FUNCTION_BLOCK "IMAC_VALVE_CALL"
TITLE =Function calls for VALVE objects
//Parameter Description for Function VALVE (FB83):
//-------------------------------------------------
//OBJ:     Ascending Object number for VALVE (1...x)
//
//RMOT:    'REMOTE'     Feedback
//                      0 = Local
//                      1 = Remote
//
//OPEN:    'OPEN'       Feedback
//                      0 = Valve is not OPEN
//                      1 = Valve is OPEN
//
//CLSD:    'CLOSED'     Feedback
//                      0 = Valve is not CLOSED
//                      1 = Valve is CLOSED
//
//ACOM:    'AUTO' Mode  Command Interface (only active, if 'REMOTE'+'AUTO')
//                      Bit  8       : Open  Command
//                      Bit  9       : Close Command
//                      Bit 11       : Lock 'Open / Close'
//                      Bit 12       : Emergency Close Command
//                      Bit 13       : Blackout Start Command
//                      Bit 14       : Pleiger 24V Valve (special function)
//
//FAUL:    'EXT. FAULT' Feedback. Function dep. on Mode Switch 'M10_ExtFaultNC':
//                      If 'M10_ExtFaultNC' = 0 :   0 = OK,    1 = Fault
//                      If 'M10_ExtFaultNC' = 1 :   0 = Fault, 1 = OK
//
//PCONF:   (leave empty, refers to local instance data in Instance DB)
//
//VOPN:    'OPEN'       Output to Valve
//                      0 = No Command
//                      1 = Open Command
//
//VCLS:    'CLOSE'      Output to Valve
//                      0 = No Command
//                      1 = Close Command
//
//STAT:    'AUTO' Mode  Status Interface
//                      Bit  8       : Valve Status Opened
//                      Bit  9       : Valve Status Closed
//                      Bit 10       : Local
//                      Bit 11       : Manual
//                      Bit 12       : Auto
//                      Bit 13       : Valve Opening
//                      Bit 14       : Valve Closing
//                      Bit 15       : Valve Alarm
//
//OSSTAT:  OS Status Word
//                      Value = 0    : Undefined
//                      Value = 1    : Opened
//                      Value = 2    : Closed
//                      Value = 3    : Opening
//                      Value = 4    : Closing
//                      Value = 5    : Undefined Position
//                      Value + 256  : Local Mode  (Offset Value)
//                      Value + 512  : Manual Mode (Offset Value)
//                      Value + 1024 : Auto Mode   (Offset Value)
//
//OSALARM: OS Alarm Word
//                      Value = 0    : Undefined
//                      Value = 1    : Normal
//                      Value = 2    : External Fault Alarm
//                      Value = 3    : Moving Alarm
//                      Value = 4    : Opening Alarm
//                      Value = 5    : Closing Alarm
//                      Value = 6    : Non-Feedback Alarm
//                      Value = 7    : Lock Start / Stop Commands
//                      Value = 8    : Emergency Off
//
//OSCOM:   OS Command Interface
//                      Bit  0       : Open   Command
//                      Bit  1       : Close  Command
//                      Bit  2       : Toggle Command
//                      Bit  7       : Reset  Command
//                      Bit  9       : Manual Command
//                      Bit 10       : Auto   Command
AUTHOR : Hottendo
FAMILY : IMAC
VERSION : 0.2


VAR
  ValveNo_001 : "IMAC_VALVE";
  ValveNo_002 : "IMAC_VALVE";
  ValveNo_003 : "IMAC_VALVE";
  ValveNo_004 : "IMAC_VALVE";
  ValveNo_005 : "IMAC_VALVE";
  ValveNo_006 : "IMAC_VALVE";
  ValveNo_007 : "IMAC_VALVE";
  ValveNo_008 : "IMAC_VALVE";
  ValveNo_009 : "IMAC_VALVE";
  ValveNo_010 : "IMAC_VALVE";
  ValveNo_011 : "IMAC_VALVE";
  ValveNo_012 : "IMAC_VALVE";
  ValveNo_013 : "IMAC_VALVE";
  ValveNo_014 : "IMAC_VALVE";
  ValveNo_015 : "IMAC_VALVE";
  ValveNo_016 : "IMAC_VALVE";
  ValveNo_017 : "IMAC_VALVE";
  ValveNo_018 : "IMAC_VALVE";
  ValveNo_019 : "IMAC_VALVE";
  ValveNo_020 : "IMAC_VALVE";
  ValveNo_021 : "IMAC_VALVE";
  ValveNo_022 : "IMAC_VALVE";
  ValveNo_023 : "IMAC_VALVE";
  ValveNo_024 : "IMAC_VALVE";
  ValveNo_025 : "IMAC_VALVE";
  ValveNo_026 : "IMAC_VALVE";
  ValveNo_027 : "IMAC_VALVE";
  ValveNo_028 : "IMAC_VALVE";
  ValveNo_029 : "IMAC_VALVE";
  ValveNo_030 : "IMAC_VALVE";
  ValveNo_031 : "IMAC_VALVE";
  ValveNo_032 : "IMAC_VALVE";
  ValveNo_033 : "IMAC_VALVE";
  ValveNo_034 : "IMAC_VALVE";
  ValveNo_035 : "IMAC_VALVE";
  ValveNo_036 : "IMAC_VALVE";
  ValveNo_037 : "IMAC_VALVE";
  ValveNo_038 : "IMAC_VALVE";
  ValveNo_039 : "IMAC_VALVE";
  ValveNo_040 : "IMAC_VALVE";
  ValveNo_041 : "IMAC_VALVE";
  ValveNo_042 : "IMAC_VALVE";
  ValveNo_043 : "IMAC_VALVE";
  ValveNo_044 : "IMAC_VALVE";
  ValveNo_045 : "IMAC_VALVE";
  ValveNo_046 : "IMAC_VALVE";
  ValveNo_047 : "IMAC_VALVE";
  ValveNo_048 : "IMAC_VALVE";
  ValveNo_049 : "IMAC_VALVE";
  ValveNo_050 : "IMAC_VALVE";
  ValveNo_051 : "IMAC_VALVE";
  ValveNo_052 : "IMAC_VALVE";
  ValveNo_053 : "IMAC_VALVE";
  ValveNo_054 : "IMAC_VALVE";
  ValveNo_055 : "IMAC_VALVE";
  ValveNo_056 : "IMAC_VALVE";
  ValveNo_057 : "IMAC_VALVE";
  ValveNo_058 : "IMAC_VALVE";
  ValveNo_059 : "IMAC_VALVE";
  ValveNo_060 : "IMAC_VALVE";
  ValveNo_061 : "IMAC_VALVE";
  ValveNo_062 : "IMAC_VALVE";
  ValveNo_063 : "IMAC_VALVE";
  ValveNo_064 : "IMAC_VALVE";
  ValveNo_065 : "IMAC_VALVE";
  ValveNo_066 : "IMAC_VALVE";
  ValveNo_067 : "IMAC_VALVE";
  ValveNo_068 : "IMAC_VALVE";
  ValveNo_069 : "IMAC_VALVE";
  ValveNo_070 : "IMAC_VALVE";
  ValveNo_071 : "IMAC_VALVE";
  ValveNo_072 : "IMAC_VALVE";
  ValveNo_073 : "IMAC_VALVE";
  ValveNo_074 : "IMAC_VALVE";
  ValveNo_075 : "IMAC_VALVE";
  ValveNo_076 : "IMAC_VALVE";
  ValveNo_077 : "IMAC_VALVE";
  ValveNo_078 : "IMAC_VALVE";
  ValveNo_079 : "IMAC_VALVE";
  ValveNo_080 : "IMAC_VALVE";
  ValveNo_081 : "IMAC_VALVE";
  ValveNo_082 : "IMAC_VALVE";
  ValveNo_083 : "IMAC_VALVE";
  ValveNo_084 : "IMAC_VALVE";
  ValveNo_085 : "IMAC_VALVE";
  ValveNo_086 : "IMAC_VALVE";
  ValveNo_087 : "IMAC_VALVE";
  ValveNo_088 : "IMAC_VALVE";
  ValveNo_089 : "IMAC_VALVE";
  ValveNo_090 : "IMAC_VALVE";
  ValveNo_091 : "IMAC_VALVE";
  ValveNo_092 : "IMAC_VALVE";
  ValveNo_093 : "IMAC_VALVE";
  ValveNo_094 : "IMAC_VALVE";
  ValveNo_095 : "IMAC_VALVE";
  ValveNo_096 : "IMAC_VALVE";
  ValveNo_097 : "IMAC_VALVE";
  ValveNo_098 : "IMAC_VALVE";
  ValveNo_099 : "IMAC_VALVE";
  ValveNo_100 : "IMAC_VALVE";
END_VAR
BEGIN
NETWORK
TITLE =VALVE Number 001

      CALL #ValveNo_001 (
           OBJ                      := 1,
           RMOT                     := E      7.6,
           OPEN                     := E      7.7,
           CLSD                     := E      8.0,
           ACOM                     := "IMAC_VALVE_I/O".VALVE_001_ACOM,
           FAUL                     := E      8.1,
           VOPN                     := A      3.6,
           VCLS                     := A      3.7,
           STAT                     := "IMAC_VALVE_I/O".VALVE_001_STAT,
           OSSTAT                   := "IMAC_VALVE_I/O".VALVE_00l_OSSTAT,
           OSALARM                  := "IMAC_VALVE_I/O".VALVE_00l_OSALARM,
           OSCOM                    := "IMAC_VALVE_I/O".VALVE_001_OSCOM);

NETWORK
TITLE =VALVE Number 002

      CALL #ValveNo_002 (
           OBJ                      := 2,
           RMOT                     := E      8.2,
           OPEN                     := E      8.3,
           CLSD                     := E      8.4,
           ACOM                     := "IMAC_VALVE_I/O".VALVE_002_ACOM,
           FAUL                     := E      8.5,
           VOPN                     := A      4.0,
           VCLS                     := A      4.1,
           STAT                     := "IMAC_VALVE_I/O".VALVE_002_STAT,
           OSSTAT                   := "IMAC_VALVE_I/O".VALVE_002_OSSTAT,
           OSALARM                  := "IMAC_VALVE_I/O".VALVE_002_OSALARM,
           OSCOM                    := "IMAC_VALVE_I/O".VALVE_002_OSCOM);

NETWORK
TITLE =VALVE Number 003

      CALL #ValveNo_003 (
           OBJ                      := 3,
           RMOT                     := E      8.6,
           OPEN                     := E      8.7,
           CLSD                     := E      9.0,
           ACOM                     := "IMAC_VALVE_I/O".VALVE_003_ACOM,
           FAUL                     := E      9.1,
           VOPN                     := A      4.2,
           VCLS                     := A      4.3,
           STAT                     := "IMAC_VALVE_I/O".VALVE_003_STAT,
           OSSTAT                   := "IMAC_VALVE_I/O".VALVE_003_OSSTAT,
           OSALARM                  := "IMAC_VALVE_I/O".VALVE_003_OSALARM,
           OSCOM                    := "IMAC_VALVE_I/O".VALVE_003_OSCOM);

NETWORK
TITLE =VALVE Number 004

//*********** END of Function Processing ! *******************************************************************
      BEA   ; // Move this Instruction down to the next Network to add one object !
//************************************************************************************************************

      CALL #ValveNo_004 (
           OBJ                      := 4,
           ACOM                     := "IMAC_VALVE_I/O".VALVE_004_ACOM,
           STAT                     := "IMAC_VALVE_I/O".VALVE_004_STAT,
           OSSTAT                   := "IMAC_VALVE_I/O".VALVE_004_OSSTAT,
           OSALARM                  := "IMAC_VALVE_I/O".VALVE_004_OSALARM,
           OSCOM                    := "IMAC_VALVE_I/O".VALVE_004_OSCOM);

NETWORK
TITLE =VALVE Number 005

      CALL #ValveNo_005 (
           OBJ                      := 5,
           ACOM                     := "IMAC_VALVE_I/O".VALVE_005_ACOM,
           STAT                     := "IMAC_VALVE_I/O".VALVE_005_STAT,
           OSSTAT                   := "IMAC_VALVE_I/O".VALVE_005_OSSTAT,
           OSALARM                  := "IMAC_VALVE_I/O".VALVE_005_OSALARM,
           OSCOM                    := "IMAC_VALVE_I/O".VALVE_005_OSCOM);

NETWORK
TITLE =VALVE Number 006

      CALL #ValveNo_006 (
           OBJ                      := 6,
           ACOM                     := "IMAC_VALVE_I/O".VALVE_006_ACOM,
           STAT                     := "IMAC_VALVE_I/O".VALVE_006_STAT,
           OSSTAT                   := "IMAC_VALVE_I/O".VALVE_006_OSSTAT,
           OSALARM                  := "IMAC_VALVE_I/O".VALVE_006_OSALARM,
           OSCOM                    := "IMAC_VALVE_I/O".VALVE_006_OSCOM);

NETWORK
TITLE =VALVE Number 007

      CALL #ValveNo_007 (
           OBJ                      := 7,
           ACOM                     := "IMAC_VALVE_I/O".VALVE_007_ACOM,
           STAT                     := "IMAC_VALVE_I/O".VALVE_007_STAT,
           OSSTAT                   := "IMAC_VALVE_I/O".VALVE_007_OSSTAT,
           OSALARM                  := "IMAC_VALVE_I/O".VALVE_007_OSALARM,
           OSCOM                    := "IMAC_VALVE_I/O".VALVE_007_OSCOM);

NETWORK
TITLE =VALVE Number 008

      CALL #ValveNo_008 (
           OBJ                      := 8,
           ACOM                     := "IMAC_VALVE_I/O".VALVE_008_ACOM,
           STAT                     := "IMAC_VALVE_I/O".VALVE_008_STAT,
           OSSTAT                   := "IMAC_VALVE_I/O".VALVE_008_OSSTAT,
           OSALARM                  := "IMAC_VALVE_I/O".VALVE_008_OSALARM,
           OSCOM                    := "IMAC_VALVE_I/O".VALVE_008_OSCOM);

NETWORK
TITLE =VALVE Number 009

      CALL #ValveNo_009 (
           OBJ                      := 9,
           ACOM                     := "IMAC_VALVE_I/O".VALVE_009_ACOM,
           STAT                     := "IMAC_VALVE_I/O".VALVE_009_STAT,
           OSSTAT                   := "IMAC_VALVE_I/O".VALVE_009_OSSTAT,
           OSALARM                  := "IMAC_VALVE_I/O".VALVE_009_OSALARM,
           OSCOM                    := "IMAC_VALVE_I/O".VALVE_009_OSCOM);

NETWORK
TITLE =VALVE Number 010

      CALL #ValveNo_010 (
           OBJ                      := 10,
           ACOM                     := "IMAC_VALVE_I/O".VALVE_010_ACOM,
           STAT                     := "IMAC_VALVE_I/O".VALVE_010_STAT,
           OSSTAT                   := "IMAC_VALVE_I/O".VALVE_010_OSSTAT,
           OSALARM                  := "IMAC_VALVE_I/O".VALVE_010_OSALARM,
           OSCOM                    := "IMAC_VALVE_I/O".VALVE_010_OSCOM);

NETWORK
TITLE =VALVE Number 011

//*********** END of Function Processing ! *******************************************************************
      BEA   ; // Move this Instruction down to the next Network to add one object !
//************************************************************************************************************

      CALL #ValveNo_011 (
           OBJ                      := 11,
           ACOM                     := "IMAC_VALVE_I/O".VALVE_011_ACOM,
           STAT                     := "IMAC_VALVE_I/O".VALVE_011_STAT,
           OSSTAT                   := "IMAC_VALVE_I/O".VALVE_01l_OSSTAT,
           OSALARM                  := "IMAC_VALVE_I/O".VALVE_01l_OSALARM,
           OSCOM                    := "IMAC_VALVE_I/O".VALVE_011_OSCOM);

NETWORK
TITLE =VALVE Number 012

      CALL #ValveNo_012 (
           OBJ                      := 12,
           ACOM                     := "IMAC_VALVE_I/O".VALVE_012_ACOM,
           STAT                     := "IMAC_VALVE_I/O".VALVE_012_STAT,
           OSSTAT                   := "IMAC_VALVE_I/O".VALVE_012_OSSTAT,
           OSALARM                  := "IMAC_VALVE_I/O".VALVE_012_OSALARM,
           OSCOM                    := "IMAC_VALVE_I/O".VALVE_012_OSCOM);

NETWORK
TITLE =VALVE Number 013

      CALL #ValveNo_013 (
           OBJ                      := 13,
           ACOM                     := "IMAC_VALVE_I/O".VALVE_013_ACOM,
           STAT                     := "IMAC_VALVE_I/O".VALVE_013_STAT,
           OSSTAT                   := "IMAC_VALVE_I/O".VALVE_013_OSSTAT,
           OSALARM                  := "IMAC_VALVE_I/O".VALVE_013_OSALARM,
           OSCOM                    := "IMAC_VALVE_I/O".VALVE_013_OSCOM);

NETWORK
TITLE =VALVE Number 014

      CALL #ValveNo_014 (
           OBJ                      := 14,
           ACOM                     := "IMAC_VALVE_I/O".VALVE_014_ACOM,
           STAT                     := "IMAC_VALVE_I/O".VALVE_014_STAT,
           OSSTAT                   := "IMAC_VALVE_I/O".VALVE_014_OSSTAT,
           OSALARM                  := "IMAC_VALVE_I/O".VALVE_014_OSALARM,
           OSCOM                    := "IMAC_VALVE_I/O".VALVE_014_OSCOM);

NETWORK
TITLE =VALVE Number 015

      CALL #ValveNo_015 (
           OBJ                      := 15,
           ACOM                     := "IMAC_VALVE_I/O".VALVE_015_ACOM,
           STAT                     := "IMAC_VALVE_I/O".VALVE_015_STAT,
           OSSTAT                   := "IMAC_VALVE_I/O".VALVE_015_OSSTAT,
           OSALARM                  := "IMAC_VALVE_I/O".VALVE_015_OSALARM,
           OSCOM                    := "IMAC_VALVE_I/O".VALVE_015_OSCOM);

NETWORK
TITLE =VALVE Number 016

      CALL #ValveNo_016 (
           OBJ                      := 16,
           ACOM                     := "IMAC_VALVE_I/O".VALVE_016_ACOM,
           STAT                     := "IMAC_VALVE_I/O".VALVE_016_STAT,
           OSSTAT                   := "IMAC_VALVE_I/O".VALVE_016_OSSTAT,
           OSALARM                  := "IMAC_VALVE_I/O".VALVE_016_OSALARM,
           OSCOM                    := "IMAC_VALVE_I/O".VALVE_016_OSCOM);

NETWORK
TITLE =VALVE Number 017

      CALL #ValveNo_017 (
           OBJ                      := 17,
           ACOM                     := "IMAC_VALVE_I/O".VALVE_017_ACOM,
           STAT                     := "IMAC_VALVE_I/O".VALVE_017_STAT,
           OSSTAT                   := "IMAC_VALVE_I/O".VALVE_017_OSSTAT,
           OSALARM                  := "IMAC_VALVE_I/O".VALVE_017_OSALARM,
           OSCOM                    := "IMAC_VALVE_I/O".VALVE_017_OSCOM);

NETWORK
TITLE =VALVE Number 018

      CALL #ValveNo_018 (
           OBJ                      := 18,
           ACOM                     := "IMAC_VALVE_I/O".VALVE_018_ACOM,
           STAT                     := "IMAC_VALVE_I/O".VALVE_018_STAT,
           OSSTAT                   := "IMAC_VALVE_I/O".VALVE_018_OSSTAT,
           OSALARM                  := "IMAC_VALVE_I/O".VALVE_018_OSALARM,
           OSCOM                    := "IMAC_VALVE_I/O".VALVE_018_OSCOM);

NETWORK
TITLE =VALVE Number 019

      CALL #ValveNo_019 (
           OBJ                      := 19,
           ACOM                     := "IMAC_VALVE_I/O".VALVE_019_ACOM,
           STAT                     := "IMAC_VALVE_I/O".VALVE_019_STAT,
           OSSTAT                   := "IMAC_VALVE_I/O".VALVE_019_OSSTAT,
           OSALARM                  := "IMAC_VALVE_I/O".VALVE_019_OSALARM,
           OSCOM                    := "IMAC_VALVE_I/O".VALVE_019_OSCOM);

NETWORK
TITLE =VALVE Number 020

      CALL #ValveNo_020 (
           OBJ                      := 20,
           ACOM                     := "IMAC_VALVE_I/O".VALVE_020_ACOM,
           STAT                     := "IMAC_VALVE_I/O".VALVE_020_STAT,
           OSSTAT                   := "IMAC_VALVE_I/O".VALVE_020_OSSTAT,
           OSALARM                  := "IMAC_VALVE_I/O".VALVE_020_OSALARM,
           OSCOM                    := "IMAC_VALVE_I/O".VALVE_020_OSCOM);

NETWORK
TITLE =VALVE Number 021

      CALL #ValveNo_021 (
           OBJ                      := 21,
           ACOM                     := "IMAC_VALVE_I/O".VALVE_021_ACOM,
           STAT                     := "IMAC_VALVE_I/O".VALVE_021_STAT,
           OSSTAT                   := "IMAC_VALVE_I/O".VALVE_02l_OSSTAT,
           OSALARM                  := "IMAC_VALVE_I/O".VALVE_02l_OSALARM,
           OSCOM                    := "IMAC_VALVE_I/O".VALVE_021_OSCOM);

NETWORK
TITLE =VALVE Number 022

      CALL #ValveNo_022 (
           OBJ                      := 22,
           ACOM                     := "IMAC_VALVE_I/O".VALVE_022_ACOM,
           STAT                     := "IMAC_VALVE_I/O".VALVE_022_STAT,
           OSSTAT                   := "IMAC_VALVE_I/O".VALVE_022_OSSTAT,
           OSALARM                  := "IMAC_VALVE_I/O".VALVE_022_OSALARM,
           OSCOM                    := "IMAC_VALVE_I/O".VALVE_022_OSCOM);

NETWORK
TITLE =VALVE Number 023

      CALL #ValveNo_023 (
           OBJ                      := 23,
           ACOM                     := "IMAC_VALVE_I/O".VALVE_023_ACOM,
           STAT                     := "IMAC_VALVE_I/O".VALVE_023_STAT,
           OSSTAT                   := "IMAC_VALVE_I/O".VALVE_023_OSSTAT,
           OSALARM                  := "IMAC_VALVE_I/O".VALVE_023_OSALARM,
           OSCOM                    := "IMAC_VALVE_I/O".VALVE_023_OSCOM);

NETWORK
TITLE =VALVE Number 024

      CALL #ValveNo_024 (
           OBJ                      := 24,
           ACOM                     := "IMAC_VALVE_I/O".VALVE_024_ACOM,
           STAT                     := "IMAC_VALVE_I/O".VALVE_024_STAT,
           OSSTAT                   := "IMAC_VALVE_I/O".VALVE_024_OSSTAT,
           OSALARM                  := "IMAC_VALVE_I/O".VALVE_024_OSALARM,
           OSCOM                    := "IMAC_VALVE_I/O".VALVE_024_OSCOM);

NETWORK
TITLE =VALVE Number 025

      CALL #ValveNo_025 (
           OBJ                      := 25,
           ACOM                     := "IMAC_VALVE_I/O".VALVE_025_ACOM,
           STAT                     := "IMAC_VALVE_I/O".VALVE_025_STAT,
           OSSTAT                   := "IMAC_VALVE_I/O".VALVE_025_OSSTAT,
           OSALARM                  := "IMAC_VALVE_I/O".VALVE_025_OSALARM,
           OSCOM                    := "IMAC_VALVE_I/O".VALVE_025_OSCOM);

NETWORK
TITLE =VALVE Number 026

      CALL #ValveNo_026 (
           OBJ                      := 26,
           ACOM                     := "IMAC_VALVE_I/O".VALVE_026_ACOM,
           STAT                     := "IMAC_VALVE_I/O".VALVE_026_STAT,
           OSSTAT                   := "IMAC_VALVE_I/O".VALVE_026_OSSTAT,
           OSALARM                  := "IMAC_VALVE_I/O".VALVE_026_OSALARM,
           OSCOM                    := "IMAC_VALVE_I/O".VALVE_026_OSCOM);

NETWORK
TITLE =VALVE Number 027

      CALL #ValveNo_027 (
           OBJ                      := 27,
           ACOM                     := "IMAC_VALVE_I/O".VALVE_027_ACOM,
           STAT                     := "IMAC_VALVE_I/O".VALVE_027_STAT,
           OSSTAT                   := "IMAC_VALVE_I/O".VALVE_027_OSSTAT,
           OSALARM                  := "IMAC_VALVE_I/O".VALVE_027_OSALARM,
           OSCOM                    := "IMAC_VALVE_I/O".VALVE_027_OSCOM);

NETWORK
TITLE =VALVE Number 028

      CALL #ValveNo_028 (
           OBJ                      := 28,
           ACOM                     := "IMAC_VALVE_I/O".VALVE_028_ACOM,
           STAT                     := "IMAC_VALVE_I/O".VALVE_028_STAT,
           OSSTAT                   := "IMAC_VALVE_I/O".VALVE_028_OSSTAT,
           OSALARM                  := "IMAC_VALVE_I/O".VALVE_028_OSALARM,
           OSCOM                    := "IMAC_VALVE_I/O".VALVE_028_OSCOM);

NETWORK
TITLE =VALVE Number 029

      CALL #ValveNo_029 (
           OBJ                      := 29,
           ACOM                     := "IMAC_VALVE_I/O".VALVE_029_ACOM,
           STAT                     := "IMAC_VALVE_I/O".VALVE_029_STAT,
           OSSTAT                   := "IMAC_VALVE_I/O".VALVE_029_OSSTAT,
           OSALARM                  := "IMAC_VALVE_I/O".VALVE_029_OSALARM,
           OSCOM                    := "IMAC_VALVE_I/O".VALVE_029_OSCOM);

NETWORK
TITLE =VALVE Number 030

      CALL #ValveNo_030 (
           OBJ                      := 30,
           ACOM                     := "IMAC_VALVE_I/O".VALVE_030_ACOM,
           STAT                     := "IMAC_VALVE_I/O".VALVE_030_STAT,
           OSSTAT                   := "IMAC_VALVE_I/O".VALVE_030_OSSTAT,
           OSALARM                  := "IMAC_VALVE_I/O".VALVE_030_OSALARM,
           OSCOM                    := "IMAC_VALVE_I/O".VALVE_030_OSCOM);

NETWORK
TITLE =VALVE Number 031

      CALL #ValveNo_031 (
           OBJ                      := 31,
           ACOM                     := "IMAC_VALVE_I/O".VALVE_031_ACOM,
           STAT                     := "IMAC_VALVE_I/O".VALVE_031_STAT,
           OSSTAT                   := "IMAC_VALVE_I/O".VALVE_03l_OSSTAT,
           OSALARM                  := "IMAC_VALVE_I/O".VALVE_03l_OSALARM,
           OSCOM                    := "IMAC_VALVE_I/O".VALVE_031_OSCOM);

NETWORK
TITLE =VALVE Number 032

      CALL #ValveNo_032 (
           OBJ                      := 32,
           ACOM                     := "IMAC_VALVE_I/O".VALVE_032_ACOM,
           STAT                     := "IMAC_VALVE_I/O".VALVE_032_STAT,
           OSSTAT                   := "IMAC_VALVE_I/O".VALVE_032_OSSTAT,
           OSALARM                  := "IMAC_VALVE_I/O".VALVE_032_OSALARM,
           OSCOM                    := "IMAC_VALVE_I/O".VALVE_032_OSCOM);

NETWORK
TITLE =VALVE Number 033

      CALL #ValveNo_033 (
           OBJ                      := 33,
           ACOM                     := "IMAC_VALVE_I/O".VALVE_033_ACOM,
           STAT                     := "IMAC_VALVE_I/O".VALVE_033_STAT,
           OSSTAT                   := "IMAC_VALVE_I/O".VALVE_033_OSSTAT,
           OSALARM                  := "IMAC_VALVE_I/O".VALVE_033_OSALARM,
           OSCOM                    := "IMAC_VALVE_I/O".VALVE_033_OSCOM);

NETWORK
TITLE =VALVE Number 034

      CALL #ValveNo_034 (
           OBJ                      := 34,
           ACOM                     := "IMAC_VALVE_I/O".VALVE_034_ACOM,
           STAT                     := "IMAC_VALVE_I/O".VALVE_034_STAT,
           OSSTAT                   := "IMAC_VALVE_I/O".VALVE_034_OSSTAT,
           OSALARM                  := "IMAC_VALVE_I/O".VALVE_034_OSALARM,
           OSCOM                    := "IMAC_VALVE_I/O".VALVE_034_OSCOM);

NETWORK
TITLE =VALVE Number 035

      CALL #ValveNo_035 (
           OBJ                      := 35,
           ACOM                     := "IMAC_VALVE_I/O".VALVE_035_ACOM,
           STAT                     := "IMAC_VALVE_I/O".VALVE_035_STAT,
           OSSTAT                   := "IMAC_VALVE_I/O".VALVE_035_OSSTAT,
           OSALARM                  := "IMAC_VALVE_I/O".VALVE_035_OSALARM,
           OSCOM                    := "IMAC_VALVE_I/O".VALVE_035_OSCOM);

NETWORK
TITLE =VALVE Number 036

      CALL #ValveNo_036 (
           OBJ                      := 36,
           ACOM                     := "IMAC_VALVE_I/O".VALVE_036_ACOM,
           STAT                     := "IMAC_VALVE_I/O".VALVE_036_STAT,
           OSSTAT                   := "IMAC_VALVE_I/O".VALVE_036_OSSTAT,
           OSALARM                  := "IMAC_VALVE_I/O".VALVE_036_OSALARM,
           OSCOM                    := "IMAC_VALVE_I/O".VALVE_036_OSCOM);

NETWORK
TITLE =VALVE Number 037

      CALL #ValveNo_037 (
           OBJ                      := 37,
           ACOM                     := "IMAC_VALVE_I/O".VALVE_037_ACOM,
           STAT                     := "IMAC_VALVE_I/O".VALVE_037_STAT,
           OSSTAT                   := "IMAC_VALVE_I/O".VALVE_037_OSSTAT,
           OSALARM                  := "IMAC_VALVE_I/O".VALVE_037_OSALARM,
           OSCOM                    := "IMAC_VALVE_I/O".VALVE_037_OSCOM);

NETWORK
TITLE =VALVE Number 038

      CALL #ValveNo_038 (
           OBJ                      := 38,
           ACOM                     := "IMAC_VALVE_I/O".VALVE_038_ACOM,
           STAT                     := "IMAC_VALVE_I/O".VALVE_038_STAT,
           OSSTAT                   := "IMAC_VALVE_I/O".VALVE_038_OSSTAT,
           OSALARM                  := "IMAC_VALVE_I/O".VALVE_038_OSALARM,
           OSCOM                    := "IMAC_VALVE_I/O".VALVE_038_OSCOM);

NETWORK
TITLE =VALVE Number 039

      CALL #ValveNo_039 (
           OBJ                      := 339,
           ACOM                     := "IMAC_VALVE_I/O".VALVE_039_ACOM,
           STAT                     := "IMAC_VALVE_I/O".VALVE_039_STAT,
           OSSTAT                   := "IMAC_VALVE_I/O".VALVE_039_OSSTAT,
           OSALARM                  := "IMAC_VALVE_I/O".VALVE_039_OSALARM,
           OSCOM                    := "IMAC_VALVE_I/O".VALVE_039_OSCOM);

NETWORK
TITLE =VALVE Number 040

      CALL #ValveNo_040 (
           OBJ                      := 40,
           ACOM                     := "IMAC_VALVE_I/O".VALVE_040_ACOM,
           STAT                     := "IMAC_VALVE_I/O".VALVE_040_STAT,
           OSSTAT                   := "IMAC_VALVE_I/O".VALVE_040_OSSTAT,
           OSALARM                  := "IMAC_VALVE_I/O".VALVE_040_OSALARM,
           OSCOM                    := "IMAC_VALVE_I/O".VALVE_040_OSCOM);

NETWORK
TITLE =VALVE Number 041

      CALL #ValveNo_041 (
           OBJ                      := 41,
           ACOM                     := "IMAC_VALVE_I/O".VALVE_041_ACOM,
           STAT                     := "IMAC_VALVE_I/O".VALVE_041_STAT,
           OSSTAT                   := "IMAC_VALVE_I/O".VALVE_04l_OSSTAT,
           OSALARM                  := "IMAC_VALVE_I/O".VALVE_04l_OSALARM,
           OSCOM                    := "IMAC_VALVE_I/O".VALVE_041_OSCOM);

NETWORK
TITLE =VALVE Number 042

      CALL #ValveNo_042 (
           OBJ                      := 42,
           ACOM                     := "IMAC_VALVE_I/O".VALVE_042_ACOM,
           STAT                     := "IMAC_VALVE_I/O".VALVE_042_STAT,
           OSSTAT                   := "IMAC_VALVE_I/O".VALVE_042_OSSTAT,
           OSALARM                  := "IMAC_VALVE_I/O".VALVE_042_OSALARM,
           OSCOM                    := "IMAC_VALVE_I/O".VALVE_042_OSCOM);

NETWORK
TITLE =VALVE Number 043

      CALL #ValveNo_043 (
           OBJ                      := 43,
           ACOM                     := "IMAC_VALVE_I/O".VALVE_043_ACOM,
           STAT                     := "IMAC_VALVE_I/O".VALVE_043_STAT,
           OSSTAT                   := "IMAC_VALVE_I/O".VALVE_043_OSSTAT,
           OSALARM                  := "IMAC_VALVE_I/O".VALVE_043_OSALARM,
           OSCOM                    := "IMAC_VALVE_I/O".VALVE_043_OSCOM);

NETWORK
TITLE =VALVE Number 044

      CALL #ValveNo_044 (
           OBJ                      := 44,
           ACOM                     := "IMAC_VALVE_I/O".VALVE_044_ACOM,
           STAT                     := "IMAC_VALVE_I/O".VALVE_044_STAT,
           OSSTAT                   := "IMAC_VALVE_I/O".VALVE_044_OSSTAT,
           OSALARM                  := "IMAC_VALVE_I/O".VALVE_044_OSALARM,
           OSCOM                    := "IMAC_VALVE_I/O".VALVE_044_OSCOM);

NETWORK
TITLE =VALVE Number 045

      CALL #ValveNo_045 (
           OBJ                      := 45,
           ACOM                     := "IMAC_VALVE_I/O".VALVE_045_ACOM,
           STAT                     := "IMAC_VALVE_I/O".VALVE_045_STAT,
           OSSTAT                   := "IMAC_VALVE_I/O".VALVE_045_OSSTAT,
           OSALARM                  := "IMAC_VALVE_I/O".VALVE_045_OSALARM,
           OSCOM                    := "IMAC_VALVE_I/O".VALVE_045_OSCOM);

NETWORK
TITLE =VALVE Number 046

      CALL #ValveNo_046 (
           OBJ                      := 46,
           ACOM                     := "IMAC_VALVE_I/O".VALVE_046_ACOM,
           STAT                     := "IMAC_VALVE_I/O".VALVE_046_STAT,
           OSSTAT                   := "IMAC_VALVE_I/O".VALVE_046_OSSTAT,
           OSALARM                  := "IMAC_VALVE_I/O".VALVE_046_OSALARM,
           OSCOM                    := "IMAC_VALVE_I/O".VALVE_046_OSCOM);

NETWORK
TITLE =VALVE Number 047

      CALL #ValveNo_047 (
           OBJ                      := 47,
           ACOM                     := "IMAC_VALVE_I/O".VALVE_047_ACOM,
           STAT                     := "IMAC_VALVE_I/O".VALVE_047_STAT,
           OSSTAT                   := "IMAC_VALVE_I/O".VALVE_047_OSSTAT,
           OSALARM                  := "IMAC_VALVE_I/O".VALVE_047_OSALARM,
           OSCOM                    := "IMAC_VALVE_I/O".VALVE_047_OSCOM);

NETWORK
TITLE =VALVE Number 048

      CALL #ValveNo_048 (
           OBJ                      := 48,
           ACOM                     := "IMAC_VALVE_I/O".VALVE_048_ACOM,
           STAT                     := "IMAC_VALVE_I/O".VALVE_048_STAT,
           OSSTAT                   := "IMAC_VALVE_I/O".VALVE_048_OSSTAT,
           OSALARM                  := "IMAC_VALVE_I/O".VALVE_048_OSALARM,
           OSCOM                    := "IMAC_VALVE_I/O".VALVE_048_OSCOM);

NETWORK
TITLE =VALVE Number 049

      CALL #ValveNo_049 (
           OBJ                      := 49,
           ACOM                     := "IMAC_VALVE_I/O".VALVE_049_ACOM,
           STAT                     := "IMAC_VALVE_I/O".VALVE_049_STAT,
           OSSTAT                   := "IMAC_VALVE_I/O".VALVE_049_OSSTAT,
           OSALARM                  := "IMAC_VALVE_I/O".VALVE_049_OSALARM,
           OSCOM                    := "IMAC_VALVE_I/O".VALVE_049_OSCOM);

NETWORK
TITLE =VALVE Number 050

      CALL #ValveNo_050 (
           OBJ                      := 50,
           ACOM                     := "IMAC_VALVE_I/O".VALVE_050_ACOM,
           STAT                     := "IMAC_VALVE_I/O".VALVE_050_STAT,
           OSSTAT                   := "IMAC_VALVE_I/O".VALVE_050_OSSTAT,
           OSALARM                  := "IMAC_VALVE_I/O".VALVE_050_OSALARM,
           OSCOM                    := "IMAC_VALVE_I/O".VALVE_050_OSCOM);

NETWORK
TITLE =VALVE Number 051

      CALL #ValveNo_051 (
           OBJ                      := 51,
           ACOM                     := "IMAC_VALVE_I/O".VALVE_051_ACOM,
           STAT                     := "IMAC_VALVE_I/O".VALVE_051_STAT,
           OSSTAT                   := "IMAC_VALVE_I/O".VALVE_05l_OSSTAT,
           OSALARM                  := "IMAC_VALVE_I/O".VALVE_05l_OSALARM,
           OSCOM                    := "IMAC_VALVE_I/O".VALVE_051_OSCOM);

NETWORK
TITLE =VALVE Number 052

      CALL #ValveNo_052 (
           OBJ                      := 52,
           ACOM                     := "IMAC_VALVE_I/O".VALVE_052_ACOM,
           STAT                     := "IMAC_VALVE_I/O".VALVE_052_STAT,
           OSSTAT                   := "IMAC_VALVE_I/O".VALVE_052_OSSTAT,
           OSALARM                  := "IMAC_VALVE_I/O".VALVE_052_OSALARM,
           OSCOM                    := "IMAC_VALVE_I/O".VALVE_052_OSCOM);

NETWORK
TITLE =VALVE Number 053

      CALL #ValveNo_053 (
           OBJ                      := 53,
           ACOM                     := "IMAC_VALVE_I/O".VALVE_053_ACOM,
           STAT                     := "IMAC_VALVE_I/O".VALVE_053_STAT,
           OSSTAT                   := "IMAC_VALVE_I/O".VALVE_053_OSSTAT,
           OSALARM                  := "IMAC_VALVE_I/O".VALVE_053_OSALARM,
           OSCOM                    := "IMAC_VALVE_I/O".VALVE_053_OSCOM);

NETWORK
TITLE =VALVE Number 054

      CALL #ValveNo_054 (
           OBJ                      := 54,
           ACOM                     := "IMAC_VALVE_I/O".VALVE_054_ACOM,
           STAT                     := "IMAC_VALVE_I/O".VALVE_054_STAT,
           OSSTAT                   := "IMAC_VALVE_I/O".VALVE_054_OSSTAT,
           OSALARM                  := "IMAC_VALVE_I/O".VALVE_054_OSALARM,
           OSCOM                    := "IMAC_VALVE_I/O".VALVE_054_OSCOM);

NETWORK
TITLE =VALVE Number 055

      CALL #ValveNo_055 (
           OBJ                      := 55,
           ACOM                     := "IMAC_VALVE_I/O".VALVE_055_ACOM,
           STAT                     := "IMAC_VALVE_I/O".VALVE_055_STAT,
           OSSTAT                   := "IMAC_VALVE_I/O".VALVE_055_OSSTAT,
           OSALARM                  := "IMAC_VALVE_I/O".VALVE_055_OSALARM,
           OSCOM                    := "IMAC_VALVE_I/O".VALVE_055_OSCOM);

NETWORK
TITLE =VALVE Number 056

      CALL #ValveNo_056 (
           OBJ                      := 56,
           ACOM                     := "IMAC_VALVE_I/O".VALVE_056_ACOM,
           STAT                     := "IMAC_VALVE_I/O".VALVE_056_STAT,
           OSSTAT                   := "IMAC_VALVE_I/O".VALVE_056_OSSTAT,
           OSALARM                  := "IMAC_VALVE_I/O".VALVE_056_OSALARM,
           OSCOM                    := "IMAC_VALVE_I/O".VALVE_056_OSCOM);

NETWORK
TITLE =VALVE Number 057

      CALL #ValveNo_057 (
           OBJ                      := 57,
           ACOM                     := "IMAC_VALVE_I/O".VALVE_057_ACOM,
           STAT                     := "IMAC_VALVE_I/O".VALVE_057_STAT,
           OSSTAT                   := "IMAC_VALVE_I/O".VALVE_057_OSSTAT,
           OSALARM                  := "IMAC_VALVE_I/O".VALVE_057_OSALARM,
           OSCOM                    := "IMAC_VALVE_I/O".VALVE_057_OSCOM);

NETWORK
TITLE =VALVE Number 058

      CALL #ValveNo_058 (
           OBJ                      := 58,
           ACOM                     := "IMAC_VALVE_I/O".VALVE_058_ACOM,
           STAT                     := "IMAC_VALVE_I/O".VALVE_058_STAT,
           OSSTAT                   := "IMAC_VALVE_I/O".VALVE_058_OSSTAT,
           OSALARM                  := "IMAC_VALVE_I/O".VALVE_058_OSALARM,
           OSCOM                    := "IMAC_VALVE_I/O".VALVE_058_OSCOM);

NETWORK
TITLE =VALVE Number 059

      CALL #ValveNo_059 (
           OBJ                      := 559,
           ACOM                     := "IMAC_VALVE_I/O".VALVE_059_ACOM,
           STAT                     := "IMAC_VALVE_I/O".VALVE_059_STAT,
           OSSTAT                   := "IMAC_VALVE_I/O".VALVE_059_OSSTAT,
           OSALARM                  := "IMAC_VALVE_I/O".VALVE_059_OSALARM,
           OSCOM                    := "IMAC_VALVE_I/O".VALVE_059_OSCOM);

NETWORK
TITLE =VALVE Number 060

      CALL #ValveNo_060 (
           OBJ                      := 60,
           ACOM                     := "IMAC_VALVE_I/O".VALVE_060_ACOM,
           STAT                     := "IMAC_VALVE_I/O".VALVE_060_STAT,
           OSSTAT                   := "IMAC_VALVE_I/O".VALVE_060_OSSTAT,
           OSALARM                  := "IMAC_VALVE_I/O".VALVE_060_OSALARM,
           OSCOM                    := "IMAC_VALVE_I/O".VALVE_060_OSCOM);

NETWORK
TITLE =VALVE Number 061

      CALL #ValveNo_061 (
           OBJ                      := 61,
           ACOM                     := "IMAC_VALVE_I/O".VALVE_061_ACOM,
           STAT                     := "IMAC_VALVE_I/O".VALVE_061_STAT,
           OSSTAT                   := "IMAC_VALVE_I/O".VALVE_06l_OSSTAT,
           OSALARM                  := "IMAC_VALVE_I/O".VALVE_06l_OSALARM,
           OSCOM                    := "IMAC_VALVE_I/O".VALVE_061_OSCOM);

NETWORK
TITLE =VALVE Number 062

      CALL #ValveNo_062 (
           OBJ                      := 62,
           ACOM                     := "IMAC_VALVE_I/O".VALVE_062_ACOM,
           STAT                     := "IMAC_VALVE_I/O".VALVE_062_STAT,
           OSSTAT                   := "IMAC_VALVE_I/O".VALVE_062_OSSTAT,
           OSALARM                  := "IMAC_VALVE_I/O".VALVE_062_OSALARM,
           OSCOM                    := "IMAC_VALVE_I/O".VALVE_062_OSCOM);

NETWORK
TITLE =VALVE Number 063

      CALL #ValveNo_063 (
           OBJ                      := 63,
           ACOM                     := "IMAC_VALVE_I/O".VALVE_063_ACOM,
           STAT                     := "IMAC_VALVE_I/O".VALVE_063_STAT,
           OSSTAT                   := "IMAC_VALVE_I/O".VALVE_063_OSSTAT,
           OSALARM                  := "IMAC_VALVE_I/O".VALVE_063_OSALARM,
           OSCOM                    := "IMAC_VALVE_I/O".VALVE_063_OSCOM);

NETWORK
TITLE =VALVE Number 064

      CALL #ValveNo_064 (
           OBJ                      := 64,
           ACOM                     := "IMAC_VALVE_I/O".VALVE_064_ACOM,
           STAT                     := "IMAC_VALVE_I/O".VALVE_064_STAT,
           OSSTAT                   := "IMAC_VALVE_I/O".VALVE_064_OSSTAT,
           OSALARM                  := "IMAC_VALVE_I/O".VALVE_064_OSALARM,
           OSCOM                    := "IMAC_VALVE_I/O".VALVE_064_OSCOM);

NETWORK
TITLE =VALVE Number 065

      CALL #ValveNo_065 (
           OBJ                      := 65,
           ACOM                     := "IMAC_VALVE_I/O".VALVE_065_ACOM,
           STAT                     := "IMAC_VALVE_I/O".VALVE_065_STAT,
           OSSTAT                   := "IMAC_VALVE_I/O".VALVE_065_OSSTAT,
           OSALARM                  := "IMAC_VALVE_I/O".VALVE_065_OSALARM,
           OSCOM                    := "IMAC_VALVE_I/O".VALVE_065_OSCOM);

NETWORK
TITLE =VALVE Number 066

      CALL #ValveNo_066 (
           OBJ                      := 66,
           ACOM                     := "IMAC_VALVE_I/O".VALVE_066_ACOM,
           STAT                     := "IMAC_VALVE_I/O".VALVE_066_STAT,
           OSSTAT                   := "IMAC_VALVE_I/O".VALVE_066_OSSTAT,
           OSALARM                  := "IMAC_VALVE_I/O".VALVE_066_OSALARM,
           OSCOM                    := "IMAC_VALVE_I/O".VALVE_066_OSCOM);

NETWORK
TITLE =VALVE Number 067

      CALL #ValveNo_067 (
           OBJ                      := 67,
           ACOM                     := "IMAC_VALVE_I/O".VALVE_067_ACOM,
           STAT                     := "IMAC_VALVE_I/O".VALVE_067_STAT,
           OSSTAT                   := "IMAC_VALVE_I/O".VALVE_067_OSSTAT,
           OSALARM                  := "IMAC_VALVE_I/O".VALVE_067_OSALARM,
           OSCOM                    := "IMAC_VALVE_I/O".VALVE_067_OSCOM);

NETWORK
TITLE =VALVE Number 068

      CALL #ValveNo_068 (
           OBJ                      := 68,
           ACOM                     := "IMAC_VALVE_I/O".VALVE_068_ACOM,
           STAT                     := "IMAC_VALVE_I/O".VALVE_068_STAT,
           OSSTAT                   := "IMAC_VALVE_I/O".VALVE_068_OSSTAT,
           OSALARM                  := "IMAC_VALVE_I/O".VALVE_068_OSALARM,
           OSCOM                    := "IMAC_VALVE_I/O".VALVE_068_OSCOM);

NETWORK
TITLE =VALVE Number 069

      CALL #ValveNo_069 (
           OBJ                      := 69,
           ACOM                     := "IMAC_VALVE_I/O".VALVE_069_ACOM,
           STAT                     := "IMAC_VALVE_I/O".VALVE_069_STAT,
           OSSTAT                   := "IMAC_VALVE_I/O".VALVE_069_OSSTAT,
           OSALARM                  := "IMAC_VALVE_I/O".VALVE_069_OSALARM,
           OSCOM                    := "IMAC_VALVE_I/O".VALVE_069_OSCOM);

NETWORK
TITLE =VALVE Number 070

      CALL #ValveNo_070 (
           OBJ                      := 70,
           ACOM                     := "IMAC_VALVE_I/O".VALVE_070_ACOM,
           STAT                     := "IMAC_VALVE_I/O".VALVE_070_STAT,
           OSSTAT                   := "IMAC_VALVE_I/O".VALVE_070_OSSTAT,
           OSALARM                  := "IMAC_VALVE_I/O".VALVE_070_OSALARM,
           OSCOM                    := "IMAC_VALVE_I/O".VALVE_070_OSCOM);

NETWORK
TITLE =VALVE Number 071

      CALL #ValveNo_071 (
           OBJ                      := 71,
           ACOM                     := "IMAC_VALVE_I/O".VALVE_071_ACOM,
           STAT                     := "IMAC_VALVE_I/O".VALVE_071_STAT,
           OSSTAT                   := "IMAC_VALVE_I/O".VALVE_07l_OSSTAT,
           OSALARM                  := "IMAC_VALVE_I/O".VALVE_07l_OSALARM,
           OSCOM                    := "IMAC_VALVE_I/O".VALVE_071_OSCOM);

NETWORK
TITLE =VALVE Number 072

      CALL #ValveNo_072 (
           OBJ                      := 72,
           ACOM                     := "IMAC_VALVE_I/O".VALVE_072_ACOM,
           STAT                     := "IMAC_VALVE_I/O".VALVE_072_STAT,
           OSSTAT                   := "IMAC_VALVE_I/O".VALVE_072_OSSTAT,
           OSALARM                  := "IMAC_VALVE_I/O".VALVE_072_OSALARM,
           OSCOM                    := "IMAC_VALVE_I/O".VALVE_072_OSCOM);

NETWORK
TITLE =VALVE Number 073

      CALL #ValveNo_073 (
           OBJ                      := 73,
           ACOM                     := "IMAC_VALVE_I/O".VALVE_073_ACOM,
           STAT                     := "IMAC_VALVE_I/O".VALVE_073_STAT,
           OSSTAT                   := "IMAC_VALVE_I/O".VALVE_073_OSSTAT,
           OSALARM                  := "IMAC_VALVE_I/O".VALVE_073_OSALARM,
           OSCOM                    := "IMAC_VALVE_I/O".VALVE_073_OSCOM);

NETWORK
TITLE =VALVE Number 074

      CALL #ValveNo_074 (
           OBJ                      := 74,
           ACOM                     := "IMAC_VALVE_I/O".VALVE_074_ACOM,
           STAT                     := "IMAC_VALVE_I/O".VALVE_074_STAT,
           OSSTAT                   := "IMAC_VALVE_I/O".VALVE_074_OSSTAT,
           OSALARM                  := "IMAC_VALVE_I/O".VALVE_074_OSALARM,
           OSCOM                    := "IMAC_VALVE_I/O".VALVE_074_OSCOM);

NETWORK
TITLE =VALVE Number 075

      CALL #ValveNo_075 (
           OBJ                      := 75,
           ACOM                     := "IMAC_VALVE_I/O".VALVE_075_ACOM,
           STAT                     := "IMAC_VALVE_I/O".VALVE_075_STAT,
           OSSTAT                   := "IMAC_VALVE_I/O".VALVE_075_OSSTAT,
           OSALARM                  := "IMAC_VALVE_I/O".VALVE_075_OSALARM,
           OSCOM                    := "IMAC_VALVE_I/O".VALVE_075_OSCOM);

NETWORK
TITLE =VALVE Number 076

      CALL #ValveNo_076 (
           OBJ                      := 76,
           ACOM                     := "IMAC_VALVE_I/O".VALVE_076_ACOM,
           STAT                     := "IMAC_VALVE_I/O".VALVE_076_STAT,
           OSSTAT                   := "IMAC_VALVE_I/O".VALVE_076_OSSTAT,
           OSALARM                  := "IMAC_VALVE_I/O".VALVE_076_OSALARM,
           OSCOM                    := "IMAC_VALVE_I/O".VALVE_076_OSCOM);

NETWORK
TITLE =VALVE Number 077

      CALL #ValveNo_077 (
           OBJ                      := 77,
           ACOM                     := "IMAC_VALVE_I/O".VALVE_077_ACOM,
           STAT                     := "IMAC_VALVE_I/O".VALVE_077_STAT,
           OSSTAT                   := "IMAC_VALVE_I/O".VALVE_077_OSSTAT,
           OSALARM                  := "IMAC_VALVE_I/O".VALVE_077_OSALARM,
           OSCOM                    := "IMAC_VALVE_I/O".VALVE_077_OSCOM);

NETWORK
TITLE =VALVE Number 078

      CALL #ValveNo_078 (
           OBJ                      := 78,
           ACOM                     := "IMAC_VALVE_I/O".VALVE_078_ACOM,
           STAT                     := "IMAC_VALVE_I/O".VALVE_078_STAT,
           OSSTAT                   := "IMAC_VALVE_I/O".VALVE_078_OSSTAT,
           OSALARM                  := "IMAC_VALVE_I/O".VALVE_078_OSALARM,
           OSCOM                    := "IMAC_VALVE_I/O".VALVE_078_OSCOM);

NETWORK
TITLE =VALVE Number 079

      CALL #ValveNo_079 (
           OBJ                      := 79,
           ACOM                     := "IMAC_VALVE_I/O".VALVE_079_ACOM,
           STAT                     := "IMAC_VALVE_I/O".VALVE_079_STAT,
           OSSTAT                   := "IMAC_VALVE_I/O".VALVE_079_OSSTAT,
           OSALARM                  := "IMAC_VALVE_I/O".VALVE_079_OSALARM,
           OSCOM                    := "IMAC_VALVE_I/O".VALVE_079_OSCOM);

NETWORK
TITLE =VALVE Number 080

      CALL #ValveNo_080 (
           OBJ                      := 80,
           ACOM                     := "IMAC_VALVE_I/O".VALVE_080_ACOM,
           STAT                     := "IMAC_VALVE_I/O".VALVE_080_STAT,
           OSSTAT                   := "IMAC_VALVE_I/O".VALVE_080_OSSTAT,
           OSALARM                  := "IMAC_VALVE_I/O".VALVE_080_OSALARM,
           OSCOM                    := "IMAC_VALVE_I/O".VALVE_080_OSCOM);

NETWORK
TITLE =VALVE Number 081

      CALL #ValveNo_081 (
           OBJ                      := 81,
           ACOM                     := "IMAC_VALVE_I/O".VALVE_081_ACOM,
           STAT                     := "IMAC_VALVE_I/O".VALVE_081_STAT,
           OSSTAT                   := "IMAC_VALVE_I/O".VALVE_08l_OSSTAT,
           OSALARM                  := "IMAC_VALVE_I/O".VALVE_08l_OSALARM,
           OSCOM                    := "IMAC_VALVE_I/O".VALVE_081_OSCOM);

NETWORK
TITLE =VALVE Number 082

      CALL #ValveNo_082 (
           OBJ                      := 82,
           ACOM                     := "IMAC_VALVE_I/O".VALVE_082_ACOM,
           STAT                     := "IMAC_VALVE_I/O".VALVE_082_STAT,
           OSSTAT                   := "IMAC_VALVE_I/O".VALVE_082_OSSTAT,
           OSALARM                  := "IMAC_VALVE_I/O".VALVE_082_OSALARM,
           OSCOM                    := "IMAC_VALVE_I/O".VALVE_082_OSCOM);

NETWORK
TITLE =VALVE Number 083

      CALL #ValveNo_083 (
           OBJ                      := 83,
           ACOM                     := "IMAC_VALVE_I/O".VALVE_083_ACOM,
           STAT                     := "IMAC_VALVE_I/O".VALVE_083_STAT,
           OSSTAT                   := "IMAC_VALVE_I/O".VALVE_083_OSSTAT,
           OSALARM                  := "IMAC_VALVE_I/O".VALVE_083_OSALARM,
           OSCOM                    := "IMAC_VALVE_I/O".VALVE_083_OSCOM);

NETWORK
TITLE =VALVE Number 084

      CALL #ValveNo_084 (
           OBJ                      := 84,
           ACOM                     := "IMAC_VALVE_I/O".VALVE_084_ACOM,
           STAT                     := "IMAC_VALVE_I/O".VALVE_084_STAT,
           OSSTAT                   := "IMAC_VALVE_I/O".VALVE_084_OSSTAT,
           OSALARM                  := "IMAC_VALVE_I/O".VALVE_084_OSALARM,
           OSCOM                    := "IMAC_VALVE_I/O".VALVE_084_OSCOM);

NETWORK
TITLE =VALVE Number 085

      CALL #ValveNo_085 (
           OBJ                      := 85,
           ACOM                     := "IMAC_VALVE_I/O".VALVE_085_ACOM,
           STAT                     := "IMAC_VALVE_I/O".VALVE_085_STAT,
           OSSTAT                   := "IMAC_VALVE_I/O".VALVE_085_OSSTAT,
           OSALARM                  := "IMAC_VALVE_I/O".VALVE_085_OSALARM,
           OSCOM                    := "IMAC_VALVE_I/O".VALVE_085_OSCOM);

NETWORK
TITLE =VALVE Number 086

      CALL #ValveNo_086 (
           OBJ                      := 86,
           ACOM                     := "IMAC_VALVE_I/O".VALVE_086_ACOM,
           STAT                     := "IMAC_VALVE_I/O".VALVE_086_STAT,
           OSSTAT                   := "IMAC_VALVE_I/O".VALVE_086_OSSTAT,
           OSALARM                  := "IMAC_VALVE_I/O".VALVE_086_OSALARM,
           OSCOM                    := "IMAC_VALVE_I/O".VALVE_086_OSCOM);

NETWORK
TITLE =VALVE Number 087

      CALL #ValveNo_087 (
           OBJ                      := 87,
           ACOM                     := "IMAC_VALVE_I/O".VALVE_087_ACOM,
           STAT                     := "IMAC_VALVE_I/O".VALVE_087_STAT,
           OSSTAT                   := "IMAC_VALVE_I/O".VALVE_087_OSSTAT,
           OSALARM                  := "IMAC_VALVE_I/O".VALVE_087_OSALARM,
           OSCOM                    := "IMAC_VALVE_I/O".VALVE_087_OSCOM);

NETWORK
TITLE =VALVE Number 088

      CALL #ValveNo_088 (
           OBJ                      := 88,
           ACOM                     := "IMAC_VALVE_I/O".VALVE_088_ACOM,
           STAT                     := "IMAC_VALVE_I/O".VALVE_088_STAT,
           OSSTAT                   := "IMAC_VALVE_I/O".VALVE_088_OSSTAT,
           OSALARM                  := "IMAC_VALVE_I/O".VALVE_088_OSALARM,
           OSCOM                    := "IMAC_VALVE_I/O".VALVE_088_OSCOM);

NETWORK
TITLE =VALVE Number 089

      CALL #ValveNo_089 (
           OBJ                      := 89,
           ACOM                     := "IMAC_VALVE_I/O".VALVE_089_ACOM,
           STAT                     := "IMAC_VALVE_I/O".VALVE_089_STAT,
           OSSTAT                   := "IMAC_VALVE_I/O".VALVE_089_OSSTAT,
           OSALARM                  := "IMAC_VALVE_I/O".VALVE_089_OSALARM,
           OSCOM                    := "IMAC_VALVE_I/O".VALVE_089_OSCOM);

NETWORK
TITLE =VALVE Number 090

      CALL #ValveNo_090 (
           OBJ                      := 90,
           ACOM                     := "IMAC_VALVE_I/O".VALVE_090_ACOM,
           STAT                     := "IMAC_VALVE_I/O".VALVE_090_STAT,
           OSSTAT                   := "IMAC_VALVE_I/O".VALVE_090_OSSTAT,
           OSALARM                  := "IMAC_VALVE_I/O".VALVE_090_OSALARM,
           OSCOM                    := "IMAC_VALVE_I/O".VALVE_090_OSCOM);

NETWORK
TITLE =VALVE Number 091

      CALL #ValveNo_091 (
           OBJ                      := 91,
           ACOM                     := "IMAC_VALVE_I/O".VALVE_091_ACOM,
           STAT                     := "IMAC_VALVE_I/O".VALVE_091_STAT,
           OSSTAT                   := "IMAC_VALVE_I/O".VALVE_09l_OSSTAT,
           OSALARM                  := "IMAC_VALVE_I/O".VALVE_09l_OSALARM,
           OSCOM                    := "IMAC_VALVE_I/O".VALVE_091_OSCOM);

NETWORK
TITLE =VALVE Number 092

      CALL #ValveNo_092 (
           OBJ                      := 92,
           ACOM                     := "IMAC_VALVE_I/O".VALVE_092_ACOM,
           STAT                     := "IMAC_VALVE_I/O".VALVE_092_STAT,
           OSSTAT                   := "IMAC_VALVE_I/O".VALVE_092_OSSTAT,
           OSALARM                  := "IMAC_VALVE_I/O".VALVE_092_OSALARM,
           OSCOM                    := "IMAC_VALVE_I/O".VALVE_092_OSCOM);

NETWORK
TITLE =VALVE Number 093

      CALL #ValveNo_093 (
           OBJ                      := 93,
           ACOM                     := "IMAC_VALVE_I/O".VALVE_093_ACOM,
           STAT                     := "IMAC_VALVE_I/O".VALVE_093_STAT,
           OSSTAT                   := "IMAC_VALVE_I/O".VALVE_093_OSSTAT,
           OSALARM                  := "IMAC_VALVE_I/O".VALVE_093_OSALARM,
           OSCOM                    := "IMAC_VALVE_I/O".VALVE_093_OSCOM);

NETWORK
TITLE =VALVE Number 094

      CALL #ValveNo_094 (
           OBJ                      := 94,
           ACOM                     := "IMAC_VALVE_I/O".VALVE_094_ACOM,
           STAT                     := "IMAC_VALVE_I/O".VALVE_094_STAT,
           OSSTAT                   := "IMAC_VALVE_I/O".VALVE_094_OSSTAT,
           OSALARM                  := "IMAC_VALVE_I/O".VALVE_094_OSALARM,
           OSCOM                    := "IMAC_VALVE_I/O".VALVE_094_OSCOM);

NETWORK
TITLE =VALVE Number 095

      CALL #ValveNo_095 (
           OBJ                      := 95,
           ACOM                     := "IMAC_VALVE_I/O".VALVE_095_ACOM,
           STAT                     := "IMAC_VALVE_I/O".VALVE_095_STAT,
           OSSTAT                   := "IMAC_VALVE_I/O".VALVE_095_OSSTAT,
           OSALARM                  := "IMAC_VALVE_I/O".VALVE_095_OSALARM,
           OSCOM                    := "IMAC_VALVE_I/O".VALVE_095_OSCOM);

NETWORK
TITLE =VALVE Number 096

      CALL #ValveNo_096 (
           OBJ                      := 96,
           ACOM                     := "IMAC_VALVE_I/O".VALVE_096_ACOM,
           STAT                     := "IMAC_VALVE_I/O".VALVE_096_STAT,
           OSSTAT                   := "IMAC_VALVE_I/O".VALVE_096_OSSTAT,
           OSALARM                  := "IMAC_VALVE_I/O".VALVE_096_OSALARM,
           OSCOM                    := "IMAC_VALVE_I/O".VALVE_096_OSCOM);

NETWORK
TITLE =VALVE Number 097

      CALL #ValveNo_097 (
           OBJ                      := 97,
           ACOM                     := "IMAC_VALVE_I/O".VALVE_097_ACOM,
           STAT                     := "IMAC_VALVE_I/O".VALVE_097_STAT,
           OSSTAT                   := "IMAC_VALVE_I/O".VALVE_097_OSSTAT,
           OSALARM                  := "IMAC_VALVE_I/O".VALVE_097_OSALARM,
           OSCOM                    := "IMAC_VALVE_I/O".VALVE_097_OSCOM);

NETWORK
TITLE =VALVE Number 098

      CALL #ValveNo_098 (
           OBJ                      := 98,
           ACOM                     := "IMAC_VALVE_I/O".VALVE_098_ACOM,
           STAT                     := "IMAC_VALVE_I/O".VALVE_098_STAT,
           OSSTAT                   := "IMAC_VALVE_I/O".VALVE_098_OSSTAT,
           OSALARM                  := "IMAC_VALVE_I/O".VALVE_098_OSALARM,
           OSCOM                    := "IMAC_VALVE_I/O".VALVE_098_OSCOM);

NETWORK
TITLE =VALVE Number 099

      CALL #ValveNo_099 (
           OBJ                      := 99,
           ACOM                     := "IMAC_VALVE_I/O".VALVE_099_ACOM,
           STAT                     := "IMAC_VALVE_I/O".VALVE_099_STAT,
           OSSTAT                   := "IMAC_VALVE_I/O".VALVE_099_OSSTAT,
           OSALARM                  := "IMAC_VALVE_I/O".VALVE_099_OSALARM,
           OSCOM                    := "IMAC_VALVE_I/O".VALVE_099_OSCOM);

NETWORK
TITLE =VALVE Number 100

      CALL #ValveNo_100 (
           OBJ                      := 100,
           ACOM                     := "IMAC_VALVE_I/O".VALVE_100_ACOM,
           STAT                     := "IMAC_VALVE_I/O".VALVE_100_STAT,
           OSSTAT                   := "IMAC_VALVE_I/O".VALVE_100_OSSTAT,
           OSALARM                  := "IMAC_VALVE_I/O".VALVE_100_OSALARM,
           OSCOM                    := "IMAC_VALVE_I/O".VALVE_100_OSCOM);

END_FUNCTION_BLOCK

